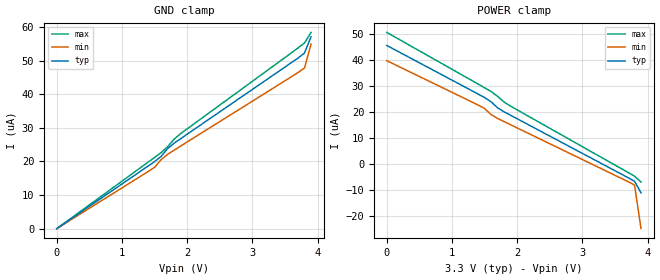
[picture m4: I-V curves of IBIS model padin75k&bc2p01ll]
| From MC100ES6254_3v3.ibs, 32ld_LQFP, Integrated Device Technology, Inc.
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|   4.0000e+00   -2.1901e-04   -2.3268e-03   -8.5970e-05
|   4.1000e+00   -7.7382e-03   -3.2912e-01   -6.2601e-04
|   4.2000e+00   -3.7622e-01   -4.7747e+01   -1.4349e-02
|   4.3000e+00   -1.8440e+01   -2.6725e+03   -3.6476e-01
|   4.4000e+00   -8.7191e+02   -7.2234e+03   -9.3138e+00
|   4.5000e+00   -4.3693e+03   -1.1774e+04   -2.3787e+02
|   4.6000e+00   -7.9281e+03   -1.6325e+04   -2.5524e+03
|   4.7000e+00   -1.1487e+04   -2.0876e+04   -5.5150e+03
|   4.8000e+00   -1.5046e+04   -2.5427e+04   -8.4775e+03
|   4.9000e+00   -1.8604e+04   -2.9978e+04   -1.1440e+04
|   5.0000e+00   -2.2163e+04   -3.4529e+04   -1.4403e+04
|   5.1000e+00   -2.5722e+04   -3.9080e+04   -1.7365e+04
|   5.2000e+00   -2.9281e+04   -4.3631e+04   -2.0328e+04
|   5.3000e+00   -3.2840e+04   -4.8182e+04   -2.3291e+04
|   5.4000e+00   -3.6398e+04   -5.2733e+04   -2.6253e+04
|   5.5000e+00   -3.9957e+04   -5.7284e+04   -2.9216e+04
|   5.6000e+00   -4.3516e+04   -6.1835e+04   -3.2178e+04
|   5.7000e+00   -4.7075e+04   -6.6386e+04   -3.5141e+04
|   5.8000e+00   -5.0634e+04   -7.0937e+04   -3.8104e+04
|   5.9000e+00   -5.4192e+04   -7.5488e+04   -4.1066e+04
|   6.0000e+00   -5.7751e+04   -8.0039e+04   -4.4029e+04
|   6.1000e+00   -6.1310e+04   -8.4590e+04   -4.6991e+04
|   6.2000e+00   -6.4869e+04   -8.9141e+04   -4.9954e+04
|   6.3000e+00   -6.8428e+04   -9.3692e+04   -5.2917e+04
|   6.4000e+00   -7.1986e+04   -9.8242e+04   -5.5879e+04
|   6.5000e+00   -7.5545e+04   -1.0279e+05   -5.8842e+04
|   6.6000e+00   -7.9104e+04   -1.0734e+05   -6.1804e+04
|..............................................................................|
| .  .  .  .  .  .  .  .  .  .  .  .  .  .  .  .  .  .  .  .  .  .  .  .  .  . |
|..............................................................................|
[Model]   padin75k&bc2p01ll
   Model_type   Input
   Polarity   Non-Inverting
   Vinl =   0.6V
   Vinh =   0.9V
   C_comp   1.0p   0.5p   1.5p
[Temperature range]   25.0   -40.0   85.0
[Voltage Range]   3.300   3.135   3.465
   |  Voltage   I(typ)   I(min)   I(max)
[GND_clamp]
|   -3.3000e+00   -7.9104e+04   -9.9835e+04   -6.6693e+04
|   -3.2000e+00   -7.5545e+04   -9.5284e+04   -6.3730e+04
|   -3.1000e+00   -7.1986e+04   -9.0733e+04   -6.0767e+04
|   -3.0000e+00   -6.8428e+04   -8.6182e+04   -5.7805e+04
|   -2.9000e+00   -6.4869e+04   -8.1632e+04   -5.4842e+04
|   -2.8000e+00   -6.1310e+04   -7.7081e+04   -5.1880e+04
|   -2.7000e+00   -5.7751e+04   -7.2530e+04   -4.8917e+04
|   -2.6000e+00   -5.4192e+04   -6.7979e+04   -4.5954e+04
|   -2.5000e+00   -5.0634e+04   -6.3428e+04   -4.2992e+04
|   -2.4000e+00   -4.7075e+04   -5.8877e+04   -4.0029e+04
|   -2.3000e+00   -4.3516e+04   -5.4326e+04   -3.7067e+04
|   -2.2000e+00   -3.9957e+04   -4.9775e+04   -3.4104e+04
|   -2.1000e+00   -3.6398e+04   -4.5224e+04   -3.1141e+04
|   -2.0000e+00   -3.2840e+04   -4.0673e+04   -2.8179e+04
|   -1.9000e+00   -2.9281e+04   -3.6122e+04   -2.5216e+04
|   -1.8000e+00   -2.5722e+04   -3.1571e+04   -2.2254e+04
|   -1.7000e+00   -2.2163e+04   -2.7020e+04   -1.9291e+04
|   -1.6000e+00   -1.8604e+04   -2.2469e+04   -1.6328e+04
|   -1.5000e+00   -1.5046e+04   -1.7918e+04   -1.3366e+04
|   -1.4000e+00   -1.1487e+04   -1.3367e+04   -1.0403e+04
|   -1.3000e+00   -7.9281e+03   -8.8163e+03   -7.4406e+03
|   -1.2000e+00   -4.3693e+03   -4.2653e+03   -4.4780e+03
|   -1.1000e+00   -8.7191e+02   -2.7260e+02   -1.5154e+03
|   -1.0000e+00   -1.8440e+01   -1.8787e+00   -7.6527e+01
|   -9.0000e-01   -3.7617e-01   -1.2959e-02   -2.9964e+00
|   -8.0000e-01   -7.6837e-03   -9.8936e-05   -1.1734e-01
|   -7.0000e-01   -1.6583e-04   -9.1041e-06   -4.6038e-03
|   -6.0000e-01   -1.1170e-05   -7.2806e-06   -1.8835e-04
|   -5.0000e-01   -6.7130e-06   -6.0637e-06   -1.4108e-05
|   -4.0000e-01   -5.3196e-06   -4.8509e-06   -5.9277e-06
|   -3.0000e-01   -3.9888e-06   -3.6382e-06   -4.2497e-06
|   -2.0000e-01   -2.6592e-06   -2.4255e-06   -2.8264e-06
|   -1.0000e-01   -1.3296e-06   -1.2127e-06   -1.4130e-06
0V        -250fA     -121.3fA   -7.564pA
1.5V      19.95uA    18.26uA    21.19uA
1.6V      21.48uA    20.52uA    22.63uA
1.7V      23.82uA    22.12uA    24.38uA
1.8V      25.43uA    23.35uA    26.64uA
1.9V      26.78uA    24.58uA    28.27uA
3.8V      52.28uA    47.85uA    55.29uA
3.9V      57.11uA    54.92uA    58.42uA
|   4.0000e+00   8.9564e-05   3.9070e-04   7.0073e-05
|   4.1000e+00   1.1895e-03   4.7653e-02   1.6060e-04
|   4.2000e+00   5.4481e-02   6.9036e+00   2.1590e-03
|   4.3000e+00   2.6663e+00   9.9777e+02   5.2838e-02
|   4.4000e+00   1.3071e+02   5.5487e+03   1.3468e+00
|   4.5000e+00   2.6945e+03   1.0100e+04   3.4393e+01
|   4.6000e+00   6.2533e+03   1.4651e+04   8.7836e+02
|   4.7000e+00   9.8121e+03   1.9202e+04   3.8402e+03
|   4.8000e+00   1.3371e+04   2.3753e+04   6.8028e+03
|   4.9000e+00   1.6930e+04   2.8303e+04   9.7654e+03
|   5.0000e+00   2.0489e+04   3.2854e+04   1.2728e+04
|   5.1000e+00   2.4047e+04   3.7405e+04   1.5691e+04
|   5.2000e+00   2.7606e+04   4.1956e+04   1.8653e+04
|   5.3000e+00   3.1165e+04   4.6507e+04   2.1616e+04
|   5.4000e+00   3.4724e+04   5.1058e+04   2.4578e+04
|   5.5000e+00   3.8282e+04   5.5609e+04   2.7541e+04
|   5.6000e+00   4.1841e+04   6.0160e+04   3.0504e+04
|   5.7000e+00   4.5400e+04   6.4711e+04   3.3466e+04
|   5.8000e+00   4.8959e+04   6.9262e+04   3.6429e+04
|   5.9000e+00   5.2518e+04   7.3813e+04   3.9391e+04
|   6.0000e+00   5.6076e+04   7.8364e+04   4.2354e+04
|   6.1000e+00   5.9635e+04   8.2915e+04   4.5317e+04
|   6.2000e+00   6.3194e+04   8.7466e+04   4.8279e+04
|   6.3000e+00   6.6753e+04   9.2017e+04   5.1242e+04
|   6.4000e+00   7.0312e+04   9.6568e+04   5.4204e+04
|   6.5000e+00   7.3870e+04   1.0112e+05   5.7167e+04
|   6.6000e+00   7.7429e+04   1.0567e+05   6.0130e+04
[POWER_clamp]
|   -3.3000e+00   7.7429e+04   9.8161e+04   6.5018e+04
|   -3.2000e+00   7.3870e+04   9.3610e+04   6.2055e+04
|   -3.1000e+00   7.0312e+04   8.9059e+04   5.9093e+04
|   -3.0000e+00   6.6753e+04   8.4508e+04   5.6130e+04
|   -2.9000e+00   6.3194e+04   7.9957e+04   5.3167e+04
|   -2.8000e+00   5.9635e+04   7.5406e+04   5.0205e+04
|   -2.7000e+00   5.6076e+04   7.0855e+04   4.7242e+04
|   -2.6000e+00   5.2518e+04   6.6304e+04   4.4280e+04
|   -2.5000e+00   4.8959e+04   6.1753e+04   4.1317e+04
|   -2.4000e+00   4.5400e+04   5.7202e+04   3.8355e+04
|   -2.3000e+00   4.1841e+04   5.2651e+04   3.5392e+04
|   -2.2000e+00   3.8282e+04   4.8100e+04   3.2429e+04
|   -2.1000e+00   3.4724e+04   4.3549e+04   2.9467e+04
|   -2.0000e+00   3.1165e+04   3.8998e+04   2.6504e+04
|   -1.9000e+00   2.7606e+04   3.4447e+04   2.3542e+04
|   -1.8000e+00   2.4047e+04   2.9896e+04   2.0579e+04
|   -1.7000e+00   2.0489e+04   2.5345e+04   1.7616e+04
|   -1.6000e+00   1.6930e+04   2.0794e+04   1.4654e+04
|   -1.5000e+00   1.3371e+04   1.6243e+04   1.1691e+04
|   -1.4000e+00   9.8121e+03   1.1693e+04   8.7285e+03
|   -1.3000e+00   6.2533e+03   7.1416e+03   5.7659e+03
|   -1.2000e+00   2.6945e+03   2.5906e+03   2.8033e+03
|   -1.1000e+00   1.3071e+02   3.9414e+01   2.8259e+02
|   -1.0000e+00   2.6663e+00   2.7172e-01   1.1065e+01
|   -9.0000e-01   5.4482e-02   1.9392e-03   4.3336e-01
|   -8.0000e-01   1.1896e-03   6.8676e-05   1.7068e-02
|   -7.0000e-01   8.9569e-05   4.8879e-05   7.5340e-04
|   -6.0000e-01   5.7110e-05   4.6884e-05   1.0100e-04
|   -5.0000e-01   5.2280e-05   4.5658e-05   6.4239e-05
|   -4.0000e-01   5.0764e-05   4.4442e-05   5.6842e-05
|   -3.0000e-01   4.9425e-05   4.3226e-05   5.4727e-05
|   -2.0000e-01   4.8092e-05   4.2011e-05   5.3270e-05
|   -1.0000e-01   4.6759e-05   4.0796e-05   5.1849e-05
0V        45.43uA    39.58uA    50.43uA
1.4V      26.78uA    22.56uA    30.62uA
1.5V      25.43uA    21.23uA    29.2uA
1.6V      23.82uA    18.89uA    27.75uA
1.7V      21.48uA    17.41uA    25.89uA
1.8V      19.95uA    16.19uA    23.68uA
1.9V      18.61uA    14.98uA    22.12uA
3.8V      -6.713uA   -8.172uA   -4.767uA
3.9V      -11.17uA   -24.91uA   -7.004uA
